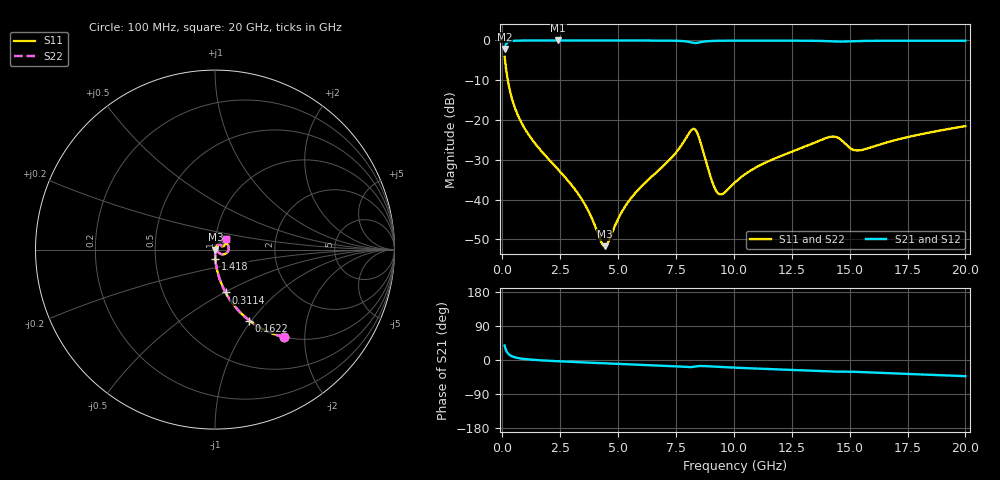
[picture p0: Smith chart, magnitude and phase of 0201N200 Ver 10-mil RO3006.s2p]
# GHz S MA R 50
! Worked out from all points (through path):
!   1601 points, 100 MHz to 20 GHz, reference 50 ohm
!   highest |S21| = -0.02 dB at 2.413 GHz (marker M1); lowest = -2.1 dB at 100 MHz (marker M2)
!   group delay of S21, straight-line fit = 6.48 ps
!   lowest |S11| = -51.7 dB at 4.428 GHz (marker M3), VSWR 1.01, Z = 50.3 - j0.0478 ohm
!   |S11| at or under -10 dB: 237.4 MHz to end of sweep
!   |S22| runs from -51.7 to -4.1 dB; largest |S21 - S12| = 0
!   S11 on the Smith chart (normalised r, x): 100 MHz: 1.00, -1.58; 162.2 MHz: 1.00, -0.98; 311.4 MHz: 1.00, -0.51; 1.418 GHz: 1.00, -0.10; 20 GHz: 1.12, +0.13
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0.1  0.6213 -51.7  0.783 38.2  0.783 38.2  0.6213 -51.7
0.1621875  0.4389 -64.2  0.8978 25.7  0.8978 25.7  0.4389 -64.2
0.3114375  0.2458 -76.2  0.9686 13.6  0.9686 13.6  0.2458 -76.2
0.721875  0.1066 -84.7  0.9933 4.7  0.9933 4.7  0.1066 -84.7
1.418375  0.05063 -88.3  0.9973 0.1  0.9973 0.1  0.05063 -88.3
2.413375  0.02387 -88.9  0.9978 -3.3  0.9978 -3.3  0.02387 -88.9
3.420812  0.01024 -83.5  0.9976 -6.1  0.9976 -6.1  0.01024 -83.5
4.42825  0.002606 -10.5  0.9973 -8.6  0.9973 -8.6  0.002606 -10.5
5.42325  0.009239 59.5  0.9967 -11.0  0.9967 -11.0  0.009239 59.5
6.741625  0.02323 63.7  0.9948 -14.4  0.9948 -14.4  0.02323 63.7
8.271437  0.07749 7.6  0.9293 -17.9  0.9293 -17.9  0.07749 7.6
8.470437  0.06308 -21.2  0.9369 -16.1  0.9369 -16.1  0.06308 -21.2
9.017687  0.01839 -33.3  0.9821 -17.1  0.9821 -17.1  0.01839 -33.3
9.278875  0.01238 -9.7  0.9875 -18.0  0.9875 -18.0  0.01238 -9.7
9.527625  0.01188 16.7  0.9901 -18.8  0.9901 -18.8  0.01188 16.7
10.05  0.01648 43.7  0.9924 -20.2  0.9924 -20.2  0.01648 43.7
11.16938  0.02737 54.3  0.9934 -23.0  0.9934 -23.0  0.02737 54.3
13.37081  0.05032 50.1  0.9885 -28.5  0.9885 -28.5  0.05032 50.1
14.35337  0.06185 31.5  0.9692 -30.6  0.9692 -30.6  0.06185 31.5
15.36081  0.04145 32.7  0.9808 -31.5  0.9808 -31.5  0.04145 32.7
16.69162  0.05321 45.8  0.9896 -34.8  0.9896 -34.8  0.05321 45.8
20  0.0839 42.8  0.9893 -42.6  0.9893 -42.6  0.0839 42.8
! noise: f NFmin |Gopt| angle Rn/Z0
0.1  0.000541  0.9212  0.3481  0.001518
2.301  0.004043  0.7756  4.522  0.003677
4.515  0.006858  0.7453  8.764  0.005379
6.729  0.01121  0.7659  12.99  0.009615
8.943  0.02662  0.8624  17.28  0.04055
11.14  0.01616  0.738  21.39  0.01193
13.36  0.02261  0.7726  25.53  0.01932
15.57  0.02994  0.7983  29.68  0.02874
17.79  0.02233  0.709  33.59  0.01387
20  0.02273  0.6859  37.47  0.01265
